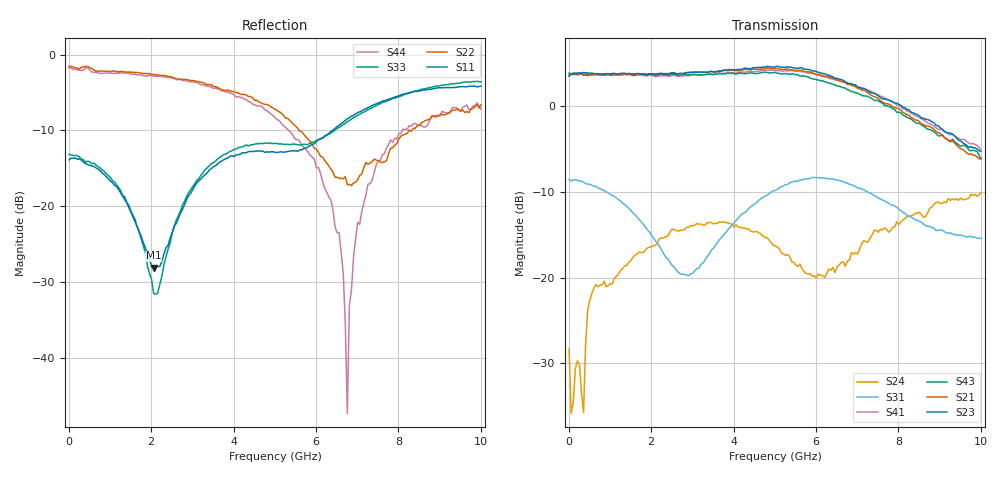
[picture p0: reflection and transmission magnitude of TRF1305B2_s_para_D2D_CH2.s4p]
! Created Thu Apr 18 16:52:43 2024
# hz S ri R 50
! 4 Port Network Data from SP1.SP block
!port1 - INP, port2 - OUTP, port3 - INM, port4 - OUTM
! freq  reS11  imS11  reS12  imS12  reS13  imS13  reS14  imS14
!  reS21  imS21  reS22  imS22  reS23  imS23  reS24  imS24
!  reS31  imS31  reS32  imS32  reS33  imS33  reS34  imS34
!  reS41  imS41  reS42  imS42  reS43  imS43  reS44  imS44
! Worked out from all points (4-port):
!   201 points, 10 MHz to 10 GHz, reference 50 ohm
!   strongest paths, dB at 10 MHz, 2.51 GHz, 5.01 GHz, 7.51 GHz, 10 GHz:
!     S23: 3.6, 3.9, 4.6, 1.2, -5.2
!     S21: 3.5, 3.9, 4.4, 0.9, -6.1
!     S43: 3.9, 3.7, 4.0, 0.7, -6.1
!     S41: 3.6, 3.6, 4.2, 1.4, -5.1
!     S31: -8.5, -18.6, -9.8, -10.7, -15.4
!     S24: -28.3, -14.3, -16.3, -14.7, -10.1
!   lowest |S11| = -28.1 dB at 2.06 GHz (marker M1), VSWR 1.08, Z = 54.1 - j0.497 ohm
!   |S11| at or under -10 dB: start of sweep to 6.399 GHz
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1e7  0.2019 -0.013  0.0081 0.00972  0.3945 -0.00216  -0.00423 0.00575
     1.497 0.023  -0.833 -0.00316  -1.519 0.0502  -0.0381 0.00628
     0.3748 0.0112  0.00923 0.0182  0.2194 -0.00732  0.00415 -0.00219
     -1.506 -0.0371  -0.0121 0.0154  1.564 -0.00028  -0.8171 0.0355
2.06e9  0.0391 -0.00458  0.0318 -0.00723  -0.0444 -0.1687  0.0512 0.00322
        0.2788 -1.516  -0.6977 0.2507  -0.1603 1.537  0.1439 0.0553
        -0.0301 -0.1676  0.0456 0.00331  0.026 -0.00579  0.0365 -0.00801
        -0.1431 1.503  0.1328 0.0455  0.2339 -1.513  -0.6767 0.2456
4.26e9  0.2126 0.0734  -0.0117 -0.0401  0.0598 0.2489  0.0406 -0.0622
        -1.617 -0.2854  -0.4221 0.3464  1.667 0.1418  0.121 -0.1536
        0.0436 0.2354  0.0381 -0.0543  0.2389 0.0721  -0.0126 -0.045
        1.574 0.1473  0.1073 -0.1166  -1.535 -0.2269  -0.3868 0.3292
5.86e9  0.2445 0.0527  -0.0288 -0.00125  0.3618 0.112  -0.0142 -0.0874
        -0.6294 1.456  -0.1739 0.2037  0.4915 -1.561  -0.0956 -0.0444
        0.3551 0.1342  -0.0117 -0.0816  0.2612 -0.00672  -0.0363 -0.000228
        0.5321 -1.476  -0.0801 -0.0343  -0.5686 1.352  -0.1012 0.1912
6.76e9  0.3762 0.034  -0.0141 0.0137  0.3351 -0.0604  -0.0532 -0.0762
        0.5147 1.239  -0.136 0.0251  -0.6331 -1.215  -0.0715 0.1022
        0.3538 -0.0484  -0.0498 -0.0735  0.3603 -0.0289  -0.017 0.0149
        -0.5368 -1.252  -0.0794 0.1006  0.4412 1.173  0.0026 0.00343
8.41e9  0.4711 -0.3257  -0.00376 -0.00398  0.1748 -0.102  -0.0946 -0.0184
        0.8231 -0.1204  -0.289 -0.1534  -0.8911 0.157  0.0201 0.2368
        0.1759 -0.1275  -0.094 -0.0172  0.4342 -0.3778  0.00102 -0.000226
        -0.8774 0.0792  0.0506 0.1861  0.8014 -0.076  -0.165 -0.3106
1e10  0.1585 -0.599  -0.019 -1.39e-05  0.1419 -0.1177  -0.0772 0.0539
      0.1933 -0.4585  -0.436 -0.1655  -0.2138 0.5036  0.1852 0.254
      0.1287 -0.1111  -0.0773 0.0568  0.0575 -0.6591  -0.0165 -0.00221
      -0.2842 0.479  0.1443 0.2104  0.1814 -0.4592  -0.3234 -0.295
